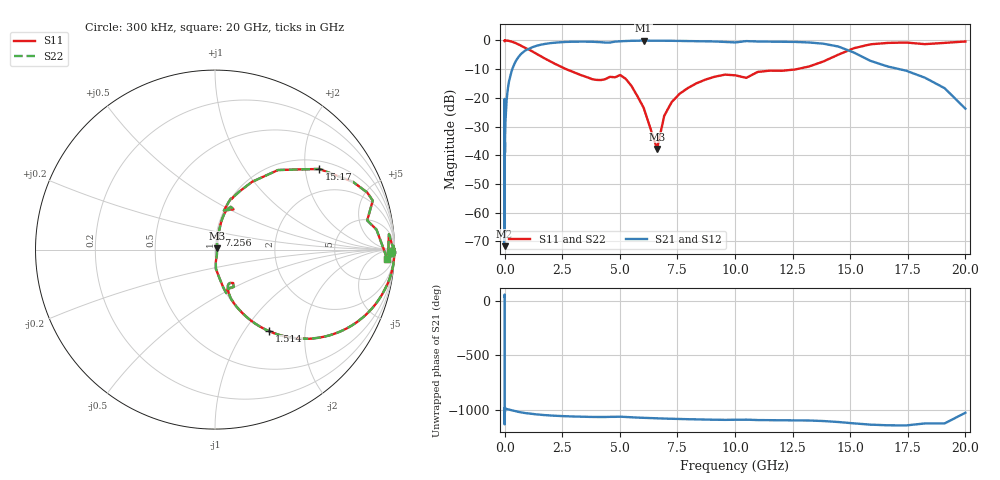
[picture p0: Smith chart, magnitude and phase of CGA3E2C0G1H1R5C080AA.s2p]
! S-parameter Generated by TDK Corporation
! Copyright(C) 2015 TDK Corporation.
! All Rights Reserved.
! TDK P/N: CGA3E2C0G1H1R5C080AA (Multilayer Ceramic Chip Capacitors)
! Property: C=1.5pF
! Size(LxWxT): 1.6x0.8x0.8mm, 0.063x0.031x0.031inches
! Model Type: s2p (Touchstone File Format Version 1.0)
! Frequency: DC=Yes Start=0.3MHz Stop=20000MHz 243points Log-sweep
! Note:
! Model Generated on Jun. 23, 2015
! Hash(MD5):
! Port Assignments:
!  1 ---| |--- 2
! Applicable Conditions:
!  Temperature = 25 degC
!  DC Bias Voltage = 0 V
!  Small Signal Operation
! Terms and conditions regarding TDK Simulation Models
! (1)This simulation model is being provided solely for informational purposes. Please refer to the specifications of the products in terms of detailed characteristics of such products.
! (2)In no event shall TDK Corporation of any of its subsidiaries be liable for any loss or damage arising, directly or indirectly,
!  From any information contained in this simulation model, including, but not limited to loss or damages arising from any inaccuracies, omissions or errors in connection with such information.
! (3)Any and all copyrights on this simulation model are owned by TDK Corporation.
!  Duplication or redistribution of this simulation model without prior written permission from TDK Corporation is prohibited.
! (4)This simulation model is subject to any modification or change without any prior notice.
! (5)Neither TDK Corporation nor any of its subsidiaries shall make any warranty, express or implied,
!  Including but not limited to the correctness, implied warranties of merchantability and fitness for a particular purpose with respect to this simulation models.
! (6)The use of this simulation model shall be deemed to have consented to the terms and conditions hereof.
# MHz S MA R 50
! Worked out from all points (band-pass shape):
!   242 points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, 300 kHz to 20 GHz, reference 50 ohm
!   highest |S21| = -0.02 dB at 6.034 GHz (marker M1); lowest = -71.6 dB at 1.506 MHz (marker M2)
!   |S21| within 3 dB of the highest: 1.033 GHz to 14.78 GHz (13.75 GHz wide, 174 % of centre)
!   lowest |S11| = -37.8 dB at 6.617 GHz (marker M3), VSWR 1.03, Z = 51.1 + j0.713 ohm
!   |S11| at or under -10 dB: 2.676 GHz to 12.67 GHz (9.997 GHz wide, 130 % of centre)
!   |S22| runs from -37.8 to 0.0 dB; largest |S21 - S12| = 3e-15
!   S11 on the Smith chart (normalised r, x): 300 kHz: 63, -49; 1.514 GHz: 1.01, -1.31; 7.256 GHz: 1.02, +0.17; 15.17 GHz: 1.22, +2.38; 20 GHz: 18, -24
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0.3  0.9803 -0.9  0.02487 37.4  0.02487 37.4  0.9803 -0.9
0.5461754  0.9994 0.0  0.003737 -80.3  0.003737 -80.3  0.9994 0.0
0.5719372  0.9737 0.0  0.0264 30.7  0.0264 30.7  0.9737 0.0
0.5989141  0.9975 -0.1  0.002774 35.1  0.002774 35.1  0.9975 -0.1
0.7201607  0.9958 1.2  0.02349 -98.4  0.02349 -98.4  0.9958 1.2
0.9067979  0.9988 -0.0  0.001239 -179.0  0.001239 -179.0  0.9988 -0.0
1.19566  0.9924 0.6  0.03049 104.3  0.03049 104.3  0.9924 0.6
1.505528  0.9998 -0.0  0.0002616 -162.0  0.0002616 -162.0  0.9998 -0.0
1.576541  0.9998 -0.3  0.004681 87.0  0.004681 87.0  0.9998 -0.3
1.985118  0.9988 -0.0  0.001337 152.4  0.001337 152.4  0.9988 -0.0
2.176801  0.9912 -0.0  0.01114 38.5  0.01114 38.5  0.9912 -0.0
2.740941  0.9996 -0.1  0.001694 77.4  0.001694 77.4  0.9996 -0.1
12.54397  0.9992 -0.7  0.01267 86.0  0.01267 86.0  0.9992 -0.7
79.26541  0.9967 -4.7  0.08124 85.3  0.08124 85.3  0.9967 -4.7
500.8786  0.8918 -26.6  0.4472 63.1  0.4472 63.1  0.8918 -26.6
1513.986  0.5465 -56.3  0.8324 33.1  0.8324 33.1  0.5465 -56.3
3165.055  0.263 -72.4  0.954 15.2  0.954 15.2  0.263 -72.4
6034.042  0.06745 -86.1  0.9977 3.9  0.9977 3.9  0.06745 -86.1
6616.689  0.0129 32.7  0.9892 -0.5  0.9892 -0.5  0.0129 32.7
7255.597  0.0849 78.0  0.9858 -4.8  0.9858 -4.8  0.0849 78.0
15168.15  0.7343 37.7  0.6144 -47.0  0.6144 -47.0  0.7343 37.7
20000  0.9604 -3.0  0.06486 50.9  0.06486 50.9  0.9604 -3.0
